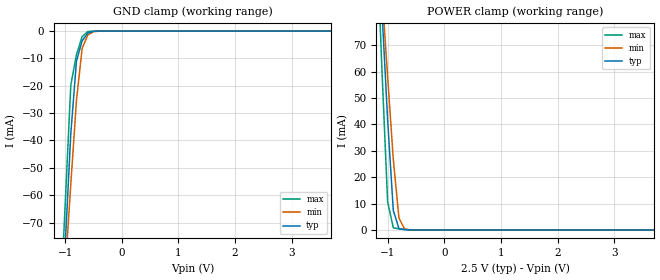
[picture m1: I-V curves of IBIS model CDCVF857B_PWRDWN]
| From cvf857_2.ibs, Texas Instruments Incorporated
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|   Model CDCVF857B_PWRDWN, update 3/2003
[Model]   CDCVF857B_PWRDWN
Model_type   Input
Polarity   Non-Inverting
Vinl = 0.7V
Vinh = 1.7V
| variable   typ   min   max
C_comp   2.0pF   1.5pF   2.5pF
[Temperature Range]   40.0   105C   0C
[Voltage range]   2.5V   2.3V   2.7V
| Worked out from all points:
|   GND clamp passes 1 mA (typ) near -0.61 V on its own axis
|   POWER clamp passes 1 mA (typ) near -0.81 V on its own axis
[GND Clamp]
|   40C:2.5V:nominal   105C:2.3V:weak   0C:2.7V:strong
|   Voltage   I(typ)   I(min)   I(max)
-2.7V     -786.6mA   -632.8mA   -974.3mA
-1.1V     -119.9mA   -120mA     -107.6mA
-900mV    -37.47mA   -55.95mA   -19.73mA
-800mV    -10.96mA   -25.29mA   -8.615mA
-700mV    -3.588mA   -6.318mA   -2.047mA
-600mV    -709.9uA   -1.433mA   -168.4uA
-500mV    -71.66uA   -235.7uA   -5.386uA
-300mV    -194.7nA   -2.508uA   -582.8pA
5.4V      137.8pA    1.376nA    112.6pA
[POWER Clamp]
|   40C:2.5V:nominal 105C:2.3V:weak   0C:2.7V:strong
|   Voltage   I(typ)   I(min)   I(max)
-2.7V     749.6mA    602.8mA    927mA
-1.2V     124.6mA    122.1mA    114.4mA
-1.1V     82.98mA    90.02mA    60.32mA
-1V       41.56mA    58.01mA    10.66mA
-900mV    7.386mA    26.7mA     830.6uA
-800mV    497uA      4.497mA    428.8uA
-700mV    137.9uA    356.4uA    187.5uA
-400mV    675.3nA    1.512uA    268.6nA
5.4V      0A         0A         0A
